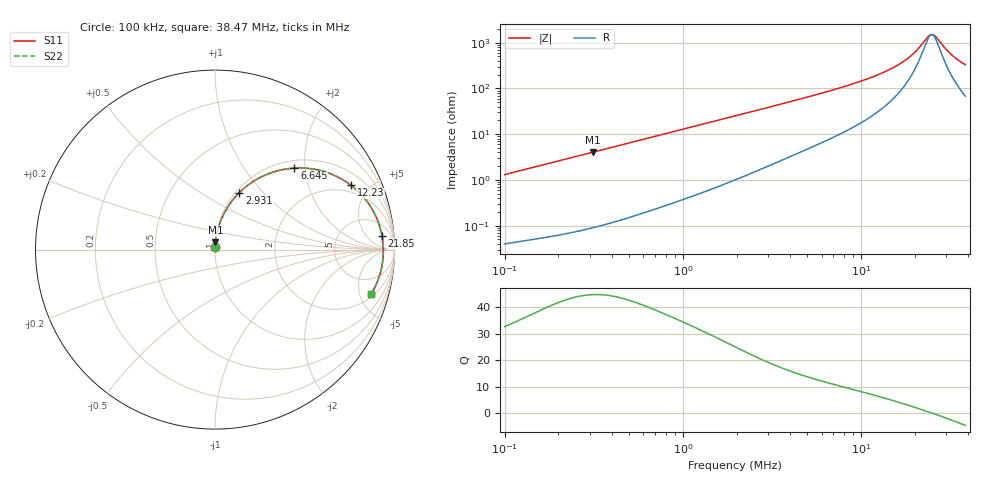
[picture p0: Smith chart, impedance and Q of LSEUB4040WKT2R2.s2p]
! LSEUB4040WKT2R2  S-PARAMETER MODEL  ( Standard Model )
! Model Generated by TAIYO YUDEN Corporation (http://www.ty-top.com)
! Version 1.0
! TAIYO YUDEN Control No. 20230502
! Copyright(c) 2023 TAIYO YUDEN CO.,LTD. All Rights Reserved.
! Product Description (link to TY-COMPAS)
! https://ds.yuden.co.jp/TYCOMPAS/or/detail?pn=LSEUB4040WKT2R2M&u=M
! Products Name : Inductors
! Characteristics :
!  Inductance : 2.2 [uH] , SRF(min) : - [Hz] , DC Resistance(max) : 0.021 [Ohm]
!  Rated Current : Saturation  7000 [mA] , Temp Rise  5300 [mA] (40 [degC])
!  Case Size : 4.0 x 4.0 / 0.157 x 0.157 [mm/inch] , Thickness : 2.0 / 0.079 [mm/inch]
!  (Conditions: Temperature = 25 [degC] , DC Bias Current = 0 [A])
! External Node Assignments :
!  1  o---GGG---o  2
! GND o---------o GND
! Frequency Range : 0.1MHz  -  38.46609MHz  [ 402 STEP ]
# MHz S RI R 50
! Freq[MHz].  S11 Real  S11 Imag  S21 Real  S21 Imag  S12 Real  S12 Imag  S22 Real  S22 Imag
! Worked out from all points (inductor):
!   401 points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, 100 kHz to 38.47 MHz, reference 50 ohm
!   read as one part in series: L = 2.07 uH near 103 kHz
!   highest Q = 44.8 at 314.5 kHz (marker M1), where L = 2.06 uH
!   self-resonance near 24.91 MHz
!   S11 on the Smith chart (normalised r, x): 100 kHz: 1.00, +0.03; 2.931 MHz: 1.04, +0.75; 6.645 MHz: 1.16, +1.75; 12.23 MHz: 1.59, +3.83; 21.85 MHz: 12, +14; 38.47 MHz: 2.36, -6.40
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0.1  0.00057 0.0131  0.9994 -0.0131  0.9994 -0.0131  0.00057 0.0131
0.27102  0.00201 0.035  0.998 -0.035  0.998 -0.035  0.00201 0.035
0.314505  0.00255 0.0405  0.9974 -0.0405  0.9974 -0.0405  0.00255 0.0405
0.734516  0.0112 0.093  0.9888 -0.093  0.9888 -0.093  0.0112 0.093
1.990681  0.0688 0.2338  0.9312 -0.2338  0.9312 -0.2338  0.0688 0.2338
2.931108  0.1351 0.3172  0.8649 -0.3172  0.8649 -0.3172  0.1351 0.3172
3.947169  0.2183 0.383  0.7817 -0.383  0.7817 -0.383  0.2183 0.383
5.315445  0.3348 0.4353  0.6652 -0.4353  0.6652 -0.4353  0.3348 0.4353
6.644771  0.442 0.4542  0.558 -0.4542  0.558 -0.4542  0.442 0.4542
9.082316  0.6077 0.4349  0.3923 -0.4349  0.3923 -0.4349  0.6077 0.4349
12.23068  0.7579 0.3581  0.2421 -0.3581  0.2421 -0.3581  0.7579 0.3581
14.40589  0.8269 0.2928  0.1731 -0.2928  0.1731 -0.2928  0.8269 0.2928
18.27861  0.9003 0.1756  0.0997 -0.1756  0.0997 -0.1756  0.9003 0.1756
19.9857  0.9182 0.1267  0.0818 -0.1267  0.0818 -0.1267  0.9182 0.1267
21.85222  0.9305 0.0761  0.0695 -0.0761  0.0695 -0.0761  0.9305 0.0761
23.89306  0.9369 0.0243  0.0631 -0.0243  0.0631 -0.0243  0.9369 0.0243
25.35844  0.938 -0.0105  0.062 0.0105  0.062 0.0105  0.938 -0.0105
26.51616  0.937 -0.0366  0.063 0.0366  0.063 0.0366  0.937 -0.0366
29.42724  0.9289 -0.0973  0.0711 0.0973  0.0711 0.0973  0.9289 -0.0973
32.17553  0.9156 -0.1484  0.0844 0.1484  0.0844 0.1484  0.9156 -0.1484
35.70792  0.8927 -0.2059  0.1073 0.2059  0.1073 0.2059  0.8927 -0.2059
38.46609  0.8715 -0.2451  0.1285 0.2451  0.1285 0.2451  0.8715 -0.2451
